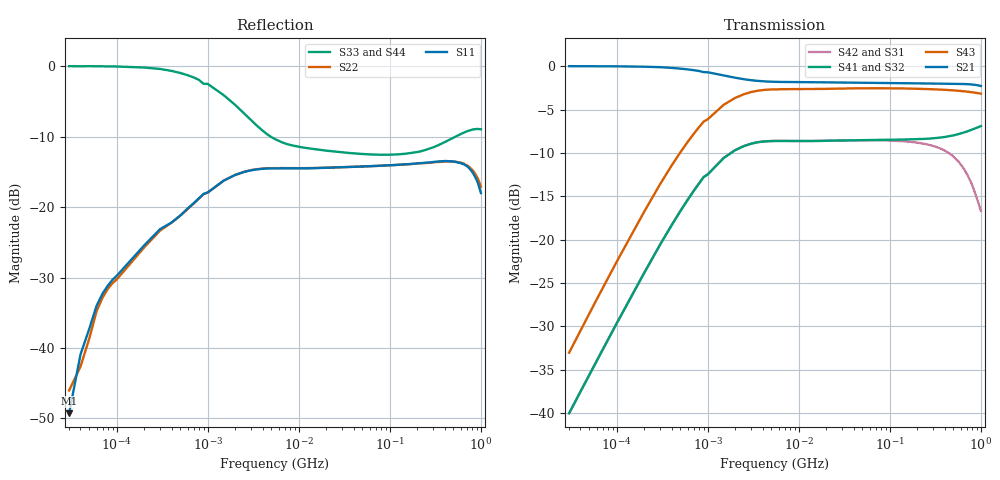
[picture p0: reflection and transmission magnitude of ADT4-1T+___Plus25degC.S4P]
!Mini-circuits Lab
!TRANSFORMER ADT4-1T+
!Tested Date: Tue Jul 10 23:49:34 2007
!Port definition PORT 1-PIN 1, PORT 2-PIN 3,PORT 3-PIN 6,PORT 4-PIN 4.
# Hz S dB R 50
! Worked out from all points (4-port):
!   1125 points, 30 kHz to 1 GHz, reference 50 ohm
!   strongest paths, dB at 30 kHz, 511.4 MHz, 567.6 MHz, 629.8 MHz, 1 GHz:
!     S21: 0.0, -2.0, -2.0, -2.0, -2.3
!     S43: -33.1, -2.8, -2.8, -2.9, -3.1
!     S41: -40.0, -7.9, -7.8, -7.7, -6.9
!     S32: -40.0, -8.0, -7.8, -7.7, -7.0
!     S42: -40.1, -10.5, -11.0, -11.6, -16.7
!     S31: -40.0, -10.6, -11.1, -11.7, -16.6
!   lowest |S11| = -49.3 dB at 30 kHz (marker M1), VSWR 1.01, Z = 49.8 - j0.234 ohm
!   |S11| at or under -10 dB: start of sweep to end of sweep
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30000  -49.29 -136.8  0.05 -0.6  -39.04 85.4  -39.10 -93.9
       0.04 -0.4  -46.04 -118.6  -39.07 -94.4  -39.11 86.1
       -40.00 87.6  -40.02 -92.2  0.04 177.9  -33.07 -91.2
       -40.04 -92.2  -40.06 87.9  -33.05 -91.5  0.02 178.2
100000  -29.75 89.6  0.03 -1.6  -28.53 80.0  -28.57 -99.6
        0.02 -1.5  -30.27 88.9  -28.54 -99.8  -28.58 80.5
        -29.63 81.3  -29.64 -98.5  -0.01 174.7  -22.57 -98.8
        -29.67 -98.5  -29.65 81.5  -22.55 -99.0  -0.04 174.9
1000000  -17.90 50.4  -0.66 -6.2  -12.08 46.4  -12.10 -133.5
         -0.67 -6.2  -17.92 50.3  -12.08 -133.6  -12.10 46.5
         -12.44 49.7  -12.43 -130.4  -2.48 150.0  -6.10 -133.5
         -12.47 -130.3  -12.45 49.7  -6.10 -133.5  -2.48 150.1
4000000  -14.54 16.5  -1.71 -4.0  -8.71 15.1  -8.72 -164.8
         -1.71 -4.0  -14.51 16.4  -8.71 -164.8  -8.72 15.2
         -8.66 15.6  -8.66 -164.4  -9.12 144.4  -2.73 -164.8
         -8.68 -164.4  -8.67 15.6  -2.73 -164.9  -9.12 144.1
3.15e7  -14.33 4.0  -1.86 -2.9  -8.53 0.4  -8.52 -179.5
        -1.86 -2.9  -14.30 4.0  -8.51 -179.7  -8.52 0.5
        -8.53 0.4  -8.53 -179.7  -12.24 164.2  -2.54 179.9
        -8.53 -179.6  -8.54 0.4  -2.54 179.9  -12.31 164.1
3.05e8  -13.56 4.6  -1.97 -20.5  -9.24 -17.9  -8.34 162.1
        -1.98 -20.6  -13.60 3.7  -8.35 160.8  -9.20 -17.7
        -9.25 -17.9  -8.30 160.3  -11.45 117.3  -2.64 157.9
        -8.29 161.5  -9.21 -17.7  -2.64 157.9  -11.42 118.2
1e9  -17.99 -21.3  -2.27 -70.2  -16.54 -24.5  -6.90 113.4
     -2.25 -70.3  -17.06 -25.1  -6.98 110.2  -16.64 -28.1
     -16.62 -24.6  -6.98 110.3  -8.93 35.3  -3.14 111.8
     -6.89 113.7  -16.67 -28.3  -3.14 111.8  -8.91 36.2
